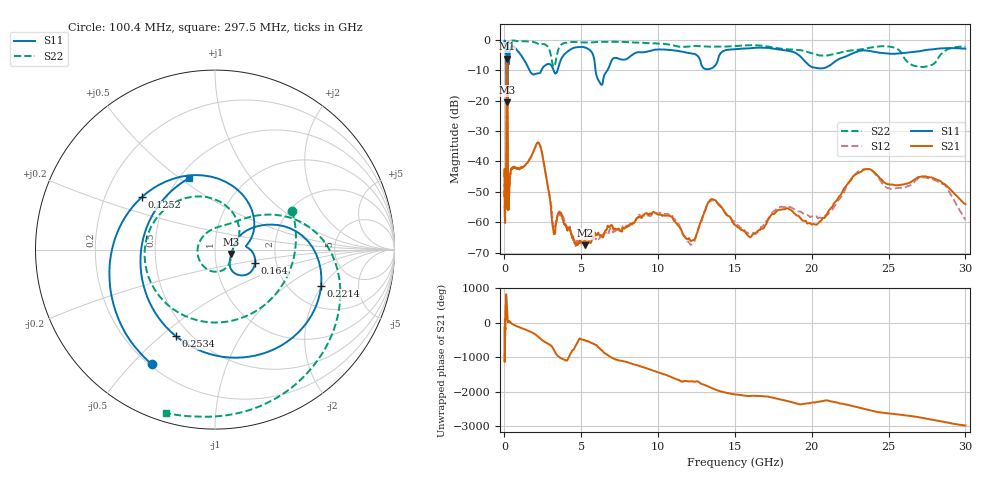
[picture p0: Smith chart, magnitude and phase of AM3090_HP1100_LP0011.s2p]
! Date/Time: Thu, Feb 28, 2019 2:06 PM
! Network Analyzer: Agilent Technologies E8364B Rev: A.07.50.67
! Sweep from 0.010 to 30.000 GHz, 1601 Points, Sweep Type: LOG
! Power Supply: 5.023 V, 0.002 A
# Hz S DB R 50
!freq MagS11 AngS11 MagS21 AngS21 MagS12 AngS12 MagS22 AngS22
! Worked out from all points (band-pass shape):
!   1601 points, 10 MHz to 30 GHz, reference 50 ohm
!   highest |S21| = -6.19 dB at 162.4 MHz (marker M1); lowest = -67.6 dB at 5.258 GHz (marker M2)
!   |S21| within 3 dB of the highest: 140.5 MHz to 192.8 MHz (52.28 MHz wide, 31.4 % of centre)
!   lowest |S11| = -20.5 dB at 191.5 MHz (marker M3), VSWR 1.21, Z = 60 - j2.93 ohm
!   |S11| at or under -10 dB: 1.625 GHz to 2.4 GHz (775.1 MHz wide, 38.5 % of centre); 3.199 GHz to 3.455 GHz (256.4 MHz wide, 7.71 % of centre); 5.926 GHz to 6.698 GHz (772.2 MHz wide, 12.2 % of centre)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
!   |S22| runs from -20.7 to -0.2 dB; largest |S21 - S12| = 0.014
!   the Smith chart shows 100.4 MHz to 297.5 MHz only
!   S11 on the Smith chart (normalised r, x): 100.4 MHz: 0.21, -0.57; 125.2 MHz: 0.36, +0.28; 164 MHz: 1.55, -0.24; 221.4 MHz: 2.93, -1.94; 253.4 MHz: 0.42, -0.56; 297.5 MHz: 0.56, +0.54
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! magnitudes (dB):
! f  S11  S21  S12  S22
! 10 MHz  -0.2  -44.8  -48.6  -0.5
! 38.04 MHz  -0.4  -58.4  -58.6  -1.3
! 100.4 MHz  -2.7  -54.5  -54.9  -6.4
! 125.2 MHz  -6.0  -25.8  -25.8  -8.1
! 144.7 MHz  -14.6  -7.7  -7.6  -19.1
! 162.4 MHz  -12.7  -6.2  -6.2  -18.3
! 164 MHz  -12.6  -6.2  -6.2  -18.2
! 191.5 MHz  -20.5  -8.8  -8.8  -17.1
! 221.4 MHz  -4.1  -45.4  -47.5  -2.6
! 253.4 MHz  -5.5  -54.6  -54.0  -0.8
! 297.5 MHz  -7.5  -51.3  -52.6  -0.4
! 550.5 MHz  -2.1  -42.0  -41.8  -0.2
! 2.084 GHz  -11.1  -34.3  -34.4  -1.0
! 3.204 GHz  -10.1  -63.6  -61.2  -8.8
! 5.258 GHz  -2.5  -67.6  -65.6  -0.8
! 6.202 GHz  -14.0  -64.3  -65.2  -0.6
! 7.926 GHz  -6.3  -61.7  -61.2  -0.7
! 12.07 GHz  -4.3  -65.8  -67.1  -2.1
! 13.68 GHz  -8.7  -52.7  -53.1  -2.2
! 16.21 GHz  -2.6  -63.9  -63.5  -1.7
! 23.48 GHz  -3.4  -42.6  -42.6  -2.9
! 30 GHz  -2.9  -54.1  -59.2  -2.2
